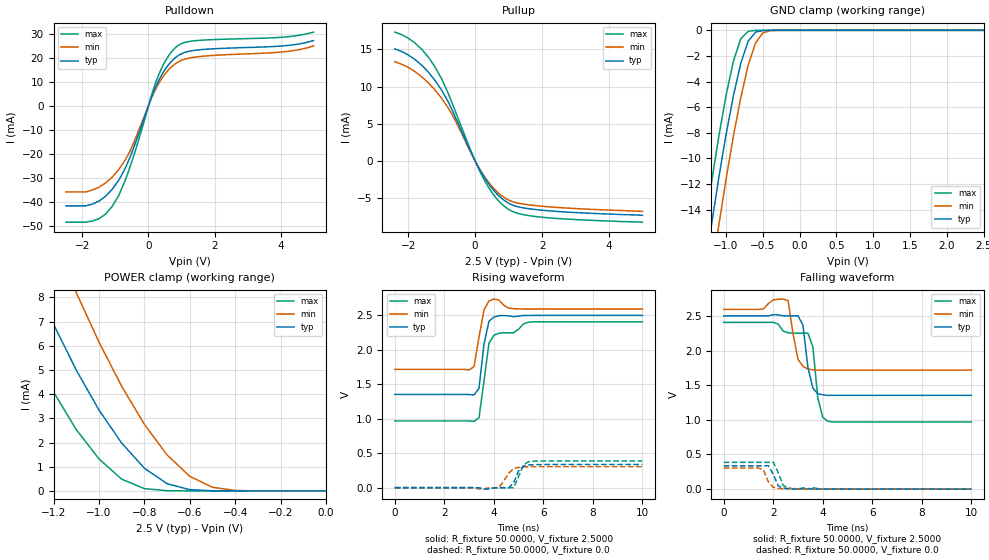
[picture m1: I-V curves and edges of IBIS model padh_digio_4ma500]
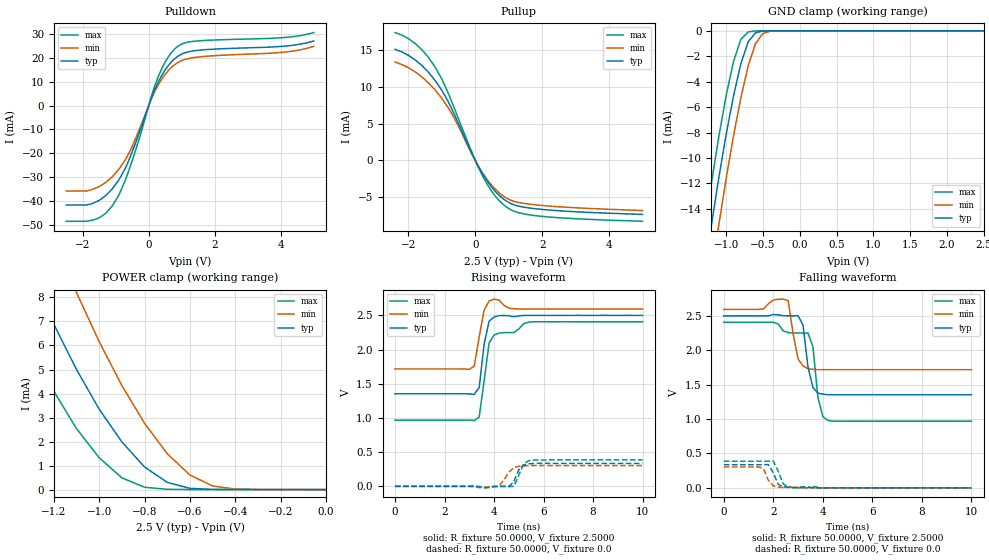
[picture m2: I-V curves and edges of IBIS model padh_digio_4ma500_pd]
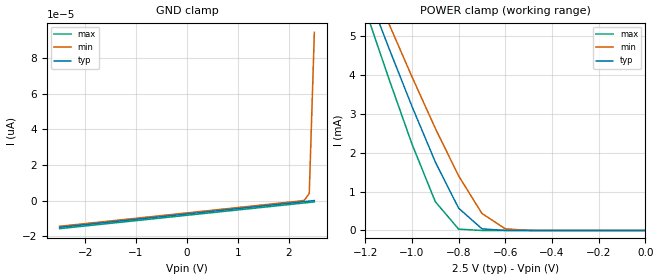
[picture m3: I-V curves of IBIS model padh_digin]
| IBIS file cs4272.ibs created by s2ibis3 verion 1.0
| North Carolina State University, ERL, 2005
[IBIS ver]   3.2
[Comment char]  |_char
[File name]   cs4272.ibs
[File Rev]   1.0B
[Date]   January 26, 2003
[Source]   HSpice Netlist
[Notes]   Rev. 1.0  1/26/2006  28-pin.  Original file.
|   Created by D. DeVries
[Copyright]   (C)opyright 2003 Cirrus Logic, Inc.  All Rights Reserved
[Component]   cs4272
[Manufacturer]  Cirrus Logic, Inc.
|   Component cs4272
[Package]
| variable   typ   min   max
R_pkg   12m   6.8m   16.1m
L_pkg   1.4n   0.713n   2.100n
C_pkg   0.27p   0.180p   0.368p
[Pin]  signal_name   model_name   R_pin   L_pin   C_pin
1   XTO   NC
2   XTI   NC
3   MCLK   padh_digio_mclk_pd
4   LRCK   padh_digio_4ma500
5   SCLK   padh_digio_4ma500
6   SDOUT   padh_digio_4ma500_pd
7   SDIN   padh_digin
8   DGND   GND
9   VD   POWER
10   VL   POWER
11   SCL_CCLK   padh_digin
12   SDA_CDIN   padh_digio_mclk
13   AD0_CSB   padh_digin
14   RSTB   padh_digin
15   VCOM   NC
16   AINA-   NC
17   AINA+   NC
18   AINB+   NC
19   AINB-   NC
20   VA   POWER
21   AGND   GND
22   FILT+   NC
23   AMUTECB   NC
24   AOUTA-   NC
25   AOUTA+   NC
26   AOUTB+   NC
27   AOUTB-   NC
28   BMUTECB   NC
| Models and submodels in the file (5): padh_digio_4ma500 (I/O), padh_digio_4ma500_pd (I/O), padh_digin (Input), padh_digio_mclk (I/O), padh_digio_mclk_pd (I/O)
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|   Model sclk
[Model]  padh_digio_4ma500
Model_type I/O
Polarity   Non-Inverting
Enable   Active-High
Vinl =   0.8000V
Vinh =   2.0000V
C_comp   5.0000pF   5.0000pF   5.0000pF
[Temperature Range]   25.0000   85.0000   -40.0000
[Voltage Range]   2.5000V   2.2500V   2.7500V
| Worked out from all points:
|   slope of the pulldown table from 0 to 0.375 V, typ, clamps not added: 30.9 ohm
|   slope of the pullup table from 0 to 0.375 V, typ, clamps not added: 129 ohm
|   GND clamp passes 1 mA (typ) near -0.71 V on its own axis
|   POWER clamp passes 1 mA (typ) near -0.81 V on its own axis
|   rising waveform, R_fixture 50.0000, V_fixture 2.5000: 20-80 % time 271ps typ, 255ps min, 349ps max; typ from 1.35 V to 2.5 V
|   rising waveform, R_fixture 50.0000, V_fixture 0.0: 20-80 % time 275ps typ, 374ps min, 276ps max; typ from 0 V to 0.336 V
|   falling waveform, R_fixture 50.0000, V_fixture 2.5000: 20-80 % time 286ps typ, 264ps min, 309ps max; typ from 2.5 V to 1.35 V
|   falling waveform, R_fixture 50.0000, V_fixture 0.0: 20-80 % time 262ps typ, 272ps min, 268ps max; typ from 0.336 V to 0 V
[Pulldown]
|Voltage   I(typ)   I(min)   I(max)
-2.5V     -41.71mA   -35.93mA   -48.52mA
-1.7V     -41.04mA   -35.15mA   -48.06mA
-1.3V     -37.72mA   -32.2mA    -45.15mA
-1.1V     -34.86mA   -29.77mA   -41.97mA
-900mV    -31.06mA   -26.62mA   -37.4mA
-600mV    -22.86mA   -20.02mA   -27.13mA
300mV     10.2mA     8.982mA    12.55mA
600mV     16.91mA    14.8mA     20.58mA
900mV     20.85mA    18.2mA     25.08mA
1.5V      23.19mA    20.36mA    27.14mA
4V        24.81mA    22.28mA    28.43mA
5V        27.08mA    24.86mA    30.63mA
[Pullup]
|Voltage   I(typ)   I(min)   I(max)
-2.4V     15.07mA    13.35mA    17.33mA
-1.8V     13.65mA    12.02mA    15.87mA
-1.2V     10.84mA    9.55mA     12.65mA
-1V       9.505mA    8.415mA    11.03mA
-600mV    5.99mA     5.516mA    6.77mA
-100mV    932.9uA    837.4uA    1.08mA
200mV     -1.679mA   -1.578mA   -1.948mA
500mV     -3.681mA   -3.422mA   -4.247mA
900mV     -5.426mA   -5.027mA   -6.222mA
1.3V      -6.208mA   -5.715mA   -7.098mA
1.9V      -6.605mA   -6.07mA    -7.546mA
5V        -7.33mA    -6.8mA     -8.26mA
[GND_clamp]
|Voltage   I(typ)   I(min)   I(max)
-2.5V     -71.95mA   -75.36mA   -70.87mA
-1.3V     -19.19mA   -23.13mA   -15.94mA
-1.2V     -15.28mA   -19.12mA   -11.98mA
-1.1V     -11.57mA   -15.28mA   -8.331mA
-1V       -8.145mA   -11.63mA   -5.085mA
-900mV    -5.12mA    -8.256mA   -2.402mA
-800mV    -2.575mA   -5.266mA   -663.9uA
-700mV    -853.9uA   -2.734mA   -79.03uA
-600mV    -146.2uA   -989.3uA   -4.169uA
-500mV    -12.66uA   -202.1uA   -123.3nA
-400mV    -717.4nA   -22.85uA   -2.473nA
2.5V      52.98pA    108.6nA    47.26pA
[POWER_clamp]
|Voltage   I(typ)   I(min)   I(max)
-2.5V     42.45mA    48.16mA    38.66mA
-1.4V     11.23mA    15.35mA    7.972mA
-1.3V     8.971mA    12.82mA    5.918mA
-1.2V     6.884mA    10.43mA    4.093mA
-1.1V     4.997mA    8.198mA    2.536mA
-1V       3.345mA    6.155mA    1.325mA
-900mV    1.981mA    4.328mA    487.2uA
-800mV    939.3uA    2.755mA    95.74uA
-700mV    299uA      1.489mA    9.484uA
-600mV    51.78uA    603.4uA    549nA
-400mV    325.5nA    21.08uA    362.3pA
0V        52.98pA    454.9pA    57.49pA
[Ramp]
| variable   typ   min   max
dV/dt_r  0.2015/0.2348n   0.1470/0.2579n   0.2770/0.1935n
dV/dt_f  0.6882/0.2375n   0.4962/0.2859n   0.9336/0.2041n
R_load = 50.0000
[Rising Waveform]
R_fixture= 50.0000
V_fixture= 2.5000
V_fixture_min= 2.7500
V_fixture_max= 2.2500
|time   V(typ)   V(min)   V(max)
0s        1.353V     1.717V     968.2mV
3ns       1.352V     1.709V     968mV
3.2ns     1.345V     1.757V     962.5mV
3.4ns     1.443V     2.187V     1.014V
3.6ns     2.079V     2.578V     1.546V
3.8ns     2.413V     2.708V     2.095V
4ns       2.475V     2.737V     2.212V
4.8ns     2.481V     2.598V     2.248V
5.4ns     2.499V     2.593V     2.401V
10ns      2.5V       2.593V     2.406V
[Rising Waveform]
R_fixture= 50.0000
V_fixture= 0.0
|time   V(typ)   V(min)   V(max)
0s        0V         0V         0V
3.2ns     253.3uV    -1.835mV   249.7uV
3.6ns     -19.91mV   -16.24mV   -22.14mV
4.2ns     -543.8uV   805.3uV    -697.7uV
4.6ns     -3.325mV   209.4mV    -1.343mV
4.8ns     69.26mV    277.8mV    -1.119mV
5ns       246mV      293.8mV    163.6mV
5.2ns     311.6mV    299.3mV    333.5mV
5.4ns     329.6mV    303.4mV    375.6mV
10ns      335.8mV    304.4mV    386.6mV
[Falling Waveform]
R_fixture= 50.0000
V_fixture= 2.5000
V_fixture_min= 2.7500
V_fixture_max= 2.2500
|time   V(typ)   V(min)   V(max)
0s        2.5V       2.593V     2.406V
2ns       2.518V     2.731V     2.407V
2.6ns     2.5V       2.72V      2.256V
3ns       2.502V     1.873V     2.25V
3.2ns     2.365V     1.772V     2.25V
3.4ns     1.758V     1.732V     2.252V
3.6ns     1.458V     1.722V     2.053V
3.8ns     1.376V     1.717V     1.315V
4.2ns     1.353V     1.717V     980.8mV
10ns      1.353V     1.717V     968.2mV
[Falling Waveform]
R_fixture= 50.0000
V_fixture= 0.0
|time   V(typ)   V(min)   V(max)
0s        335.8mV    304.4mV    386.6mV
1.4ns     335.7mV    305.1mV    386.6mV
1.6ns     335.8mV    280.7mV    386.6mV
1.8ns     338.5mV    106.8mV    386.7mV
2ns       217.7mV    26.89mV    390.7mV
2.2ns     47.85mV    11.02mV    237.9mV
2.4ns     15.93mV    4.686mV    54.05mV
2.8ns     1.992mV    11.14mV    5.021mV
3.6ns     1.596mV    -77.19uV   21.67mV
10ns      14.98uV    32.38uV    3.292uV
|   Model sclk
[Model]  padh_digio_4ma500_pd
Model_type I/O
Polarity   Non-Inverting
Enable   Active-High
Vinl =   0.8000V
Vinh =   2.0000V
C_comp   5.0000pF   5.0000pF   5.0000pF
[Temperature Range]   25.0000   85.0000   -40.0000
[Voltage Range]   2.5000V   2.2500V   2.7500V
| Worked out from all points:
|   slope of the pulldown table from 0 to 0.375 V, typ, clamps not added: 30.9 ohm
|   slope of the pullup table from 0 to 0.375 V, typ, clamps not added: 129 ohm
|   GND clamp passes 1 mA (typ) near -0.71 V on its own axis
|   POWER clamp passes 1 mA (typ) near -0.81 V on its own axis
|   rising waveform, R_fixture 50.0000, V_fixture 2.5000: 20-80 % time 270ps typ, 255ps min, 348ps max; typ from 1.35 V to 2.5 V
|   rising waveform, R_fixture 50.0000, V_fixture 0.0: 20-80 % time 277ps typ, 377ps min, 277ps max; typ from 0 V to 0.336 V
|   falling waveform, R_fixture 50.0000, V_fixture 2.5000: 20-80 % time 286ps typ, 264ps min, 310ps max; typ from 2.5 V to 1.35 V
|   falling waveform, R_fixture 50.0000, V_fixture 0.0: 20-80 % time 262ps typ, 275ps min, 269ps max; typ from 0.336 V to 0 V
[Pulldown]
|Voltage   I(typ)   I(min)   I(max)
-2.5V     -41.71mA   -35.85mA   -48.53mA
-1.7V     -41.04mA   -35.15mA   -48.06mA
-1.3V     -37.71mA   -32.21mA   -45.15mA
-1.1V     -34.86mA   -29.77mA   -41.98mA
-900mV    -31.06mA   -26.63mA   -37.41mA
-600mV    -22.87mA   -20.02mA   -27.12mA
300mV     10.2mA     8.981mA    12.55mA
600mV     16.91mA    14.8mA     20.59mA
900mV     20.85mA    18.2mA     25.08mA
1.5V      23.19mA    20.36mA    27.14mA
4V        24.81mA    22.28mA    28.43mA
5V        27.08mA    24.86mA    30.63mA
[Pullup]
|Voltage   I(typ)   I(min)   I(max)
-2.4V     15.07mA    13.35mA    17.34mA
-1.8V     13.65mA    12.02mA    15.87mA
-1.2V     10.85mA    9.55mA     12.65mA
-1V       9.504mA    8.414mA    11.03mA
-600mV    5.991mA    5.515mA    6.769mA
-100mV    932.8uA    837.4uA    1.08mA
200mV     -1.679mA   -1.577mA   -1.948mA
500mV     -3.681mA   -3.422mA   -4.247mA
900mV     -5.426mA   -5.026mA   -6.222mA
1.3V      -6.208mA   -5.715mA   -7.098mA
1.9V      -6.605mA   -6.07mA    -7.547mA
5V        -7.32mA    -6.8mA     -8.26mA
[GND_clamp]
|Voltage   I(typ)   I(min)   I(max)
-2.5V     -71.96mA   -75.36mA   -70.87mA
-1.3V     -19.2mA    -23.13mA   -15.94mA
-1.2V     -15.29mA   -19.12mA   -11.99mA
-1.1V     -11.57mA   -15.28mA   -8.335mA
-1V       -8.148mA   -11.63mA   -5.089mA
-900mV    -5.123mA   -8.258mA   -2.405mA
-800mV    -2.577mA   -5.268mA   -666.8uA
-700mV    -855.9uA   -2.736mA   -81.48uA
-600mV    -147.9uA   -990.8uA   -6.24uA
-500mV    -14.07uA   -203.3uA   -1.822uA
-400mV    -1.823uA   -23.83uA   -1.337uA
2.5V      1.678uA    1.494uA    2.16uA
[POWER_clamp]
|Voltage   I(typ)   I(min)   I(max)
-2.5V     42.45mA    48.16mA    38.67mA
-1.4V     11.23mA    15.35mA    7.974mA
-1.3V     8.973mA    12.82mA    5.921mA
-1.2V     6.885mA    10.43mA    4.095mA
-1.1V     4.999mA    8.2mA      2.538mA
-1V       3.346mA    6.156mA    1.327mA
-900mV    1.983mA    4.329mA    489.3uA
-800mV    941uA      2.756mA    97.9uA
-700mV    300.6uA    1.491mA    11.65uA
-600mV    53.46uA    604.7uA    2.713uA
-400mV    2.005uA    22.46uA    2.163uA
0V        0A         0A         0A
[Ramp]
| variable   typ   min   max
dV/dt_r  0.2014/0.2356n   0.1470/0.2600n   0.2770/0.1953n
dV/dt_f  0.6876/0.2372n   0.4962/0.2859n   0.9336/0.2044n
R_load = 50.0000
[Rising Waveform]
R_fixture= 50.0000
V_fixture= 2.5000
V_fixture_min= 2.7500
V_fixture_max= 2.2500
|time   V(typ)   V(min)   V(max)
0s        1.353V     1.717V     968.1mV
3ns       1.352V     1.709V     968mV
3.2ns     1.345V     1.757V     962.5mV
3.4ns     1.443V     2.186V     1.014V
3.6ns     2.079V     2.578V     1.544V
3.8ns     2.413V     2.708V     2.095V
4ns       2.475V     2.737V     2.212V
4.8ns     2.481V     2.597V     2.248V
5.4ns     2.499V     2.593V     2.401V
10ns      2.499V     2.593V     2.406V
[Rising Waveform]
R_fixture= 50.0000
V_fixture= 0.0
|time   V(typ)   V(min)   V(max)
0s        0V         0V         0V
3.2ns     251.4uV    -1.817mV   247.9uV
3.6ns     -19.79mV   -16.25mV   -22.02mV
4.2ns     -588.1uV   760.5uV    -714.8uV
4.6ns     -3.292mV   207.5mV    -1.331mV
4.8ns     68.29mV    276.4mV    -1.123mV
5ns       244mV      293.3mV    161.8mV
5.2ns     310.6mV    299.1mV    331.8mV
5.4ns     328.7mV    303.4mV    375.2mV
10ns      335.7mV    304.4mV    386.5mV
[Falling Waveform]
R_fixture= 50.0000
V_fixture= 2.5000
V_fixture_min= 2.7500
V_fixture_max= 2.2500
|time   V(typ)   V(min)   V(max)
0s        2.499V     2.593V     2.406V
2ns       2.518V     2.731V     2.406V
2.6ns     2.5V       2.72V      2.256V
3ns       2.502V     1.873V     2.25V
3.2ns     2.365V     1.772V     2.249V
3.4ns     1.758V     1.732V     2.251V
3.6ns     1.458V     1.722V     2.053V
3.8ns     1.376V     1.717V     1.316V
4.2ns     1.353V     1.717V     981mV
10ns      1.353V     1.717V     968.2mV
[Falling Waveform]
R_fixture= 50.0000
V_fixture= 0.0
|time   V(typ)   V(min)   V(max)
0s        335.7mV    304.4mV    386.6mV
1.4ns     335.7mV    305.1mV    386.6mV
1.6ns     335.8mV    281mV      386.5mV
1.8ns     338.4mV    109.1mV    386.6mV
2ns       219.3mV    28.14mV    390.7mV
2.2ns     49.57mV    11.46mV    239.6mV
2.4ns     16.5mV     4.88mV     55.66mV
2.8ns     2.08mV     11.15mV    5.2mV
3.6ns     1.627mV    -82.14uV   21.54mV
10ns      15.77uV    30.01uV    2.768uV
|   Model padh_digin
[Model]  padh_digin
Model_type Input
Vinl =   0.8000V
Vinh =   2.0000V
C_comp   5.0000pF   5.0000pF   5.0000pF
[Temperature Range]   25.0000   85.0000   -40.0000
[Voltage Range]   2.5000V   2.2500V   2.7500V
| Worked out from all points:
|   POWER clamp passes 1 mA (typ) near -0.84 V on its own axis
[GND_clamp]
|Voltage   I(typ)   I(min)   I(max)
-2.5V     -15pA      -14.42pA   -15.75pA
2.3V      -600.1fA   122.4fA    -1.35pA
2.4V      -300.1fA   3.964pA    -1.05pA
2.5V      0A         94.27pA    -750fA
[POWER_clamp]
|Voltage   I(typ)   I(min)   I(max)
-2.5V     27.55mA    25.88mA    29.93mA
-1.2V     6.274mA    6.747mA    5.694mA
-1.1V     4.711mA    5.337mA    3.925mA
-1V       3.195mA    3.956mA    2.226mA
-900mV    1.764mA    2.629mA    741.3uA
-800mV    572.3uA    1.403mA    34.11uA
-700mV    41.8uA     437uA      266.3nA
-600mV    967.8nA    41.61uA    1.853nA
-500mV    19.92nA    1.821uA    14.35pA
0V        0A         0A         0A
